(* Logix 5000 DataType export VMAC_DATA_INTERNAL; software revision 30.00 *)

TYPE Std_DiscreteAlarm :   // ALARM RESET
STRUCT
   AckC : BOOL;   // ALARM ACKNOWLEDGE
   LatchA : BOOL;   // ALARM LATCH
   DetectS : BOOL;   // ALARM DETECT
   BitS : BOOL;   // ALARM MISCOMPARE
   InhibitC : BOOL;   // ALARM INHIBIT
   Tmr : TIMER;   // ALARM Timer
END_STRUCT
END_TYPE

TYPE VMAC_DATA_INTERNAL :
STRUCT
   VMACOK : BOOL;
   CommsOK : BOOL;
   KeyOK : BOOL;
   KsInUse : BOOL;
   KsPrimeInUse : BOOL;
   EntryStatus : INT;
   NodeID : DINT;
   DestinationID : DINT;
   Counter : LINT;
   LastCounter : LINT;
   KeyID : LINT;
   VMAC_KEY : DINT[8];
   VMAC_CALC : DINT[8];
   VMAC_INPUT : DINT[8];
   DATA_INPUT : DINT[1600];
   DATA_VERIFIED : DINT[1600];
   VMAC_CTRL : VMAC;
   KeyAlarm : Std_DiscreteAlarm;
   ReplayAlarm : Std_DiscreteAlarm;
   InvalidAlarm : Std_DiscreteAlarm;
   NodeAlarm : Std_DiscreteAlarm;
   DestinationAlarm : Std_DiscreteAlarm;
   L_LES : L_LES;
   L_EQU : L_EQU;
   CommsTimer : TIMER;
END_STRUCT
END_TYPE

ADD_ON_INSTRUCTION D_SHR   (* revision 1.0 20170524, vendor Kenneth A. Fischer *)
// DINT bit shift right of the 32-bit argument Inp_A by Inp_B bits with paddding by zeros on the right
// Revision note:
// Rev1.0: 20170524 - Initial Release
VAR_IN_OUT
   Inp_A : DINT; {required}   // 64-bit Integer to be right circular rotated
END_VAR
VAR_INPUT
   Inp_B : INT; {required}   // Number of bits to shift
END_VAR
VAR_IN_OUT
   Out : DINT; {required}   // Result
END_VAR
VAR
   BSR_Cntrl : CONTROL := (LEN := 32);
   ONS : BOOL;
   Source_Bit : BOOL;
   Wrk_InpA : DINT[2];
END_VAR

ROUTINE Logic   (* ladder *)
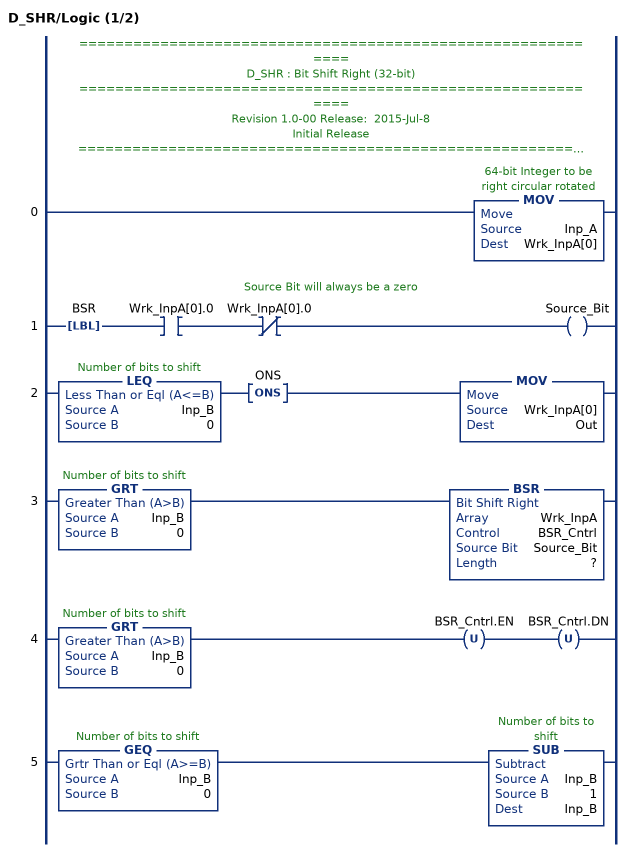
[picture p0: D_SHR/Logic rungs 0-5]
   // ============================================================
   // D_SHR : Bit Shift Right (32-bit)
   // ============================================================
   // Revision 1.0-00 Release:  2015-Jul-8
   // Initial Release
   // ============================================================
   // Performs a right bit shift of the 32-bit argument Inp_A by the
   // number of bits defined in the 16-bit argument Inp_B, with padding by zeros.
   0: MOV(Inp_A,Wrk_InpA[0]);
   // Source Bit will always be a zero
   1: LBL(BSR)XIC(Wrk_InpA[0].0)XIO(Wrk_InpA[0].0)OTE(Source_Bit);
   2: LEQ(Inp_B,0)ONS(ONS)MOV(Wrk_InpA[0],Out);
   3: GRT(Inp_B,0)BSR(Wrk_InpA,BSR_Cntrl,Source_Bit,?);
   4: GRT(Inp_B,0)OTU(BSR_Cntrl.EN)OTU(BSR_Cntrl.DN);
   5: GEQ(Inp_B,0)SUB(Inp_B,1,Inp_B);
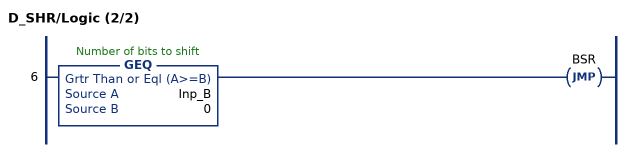
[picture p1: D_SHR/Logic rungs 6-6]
   6: GEQ(Inp_B,0)JMP(BSR);
END_ROUTINE
END_ADD_ON_INSTRUCTION

ADD_ON_INSTRUCTION D_ROTR   (* revision 1.0 20170524, vendor Kenneth A. Fischer *)
// DINT circular right shift (rotation) of the 32-bit argument Inp_A by Inp_B bits
// Revision note:
// Rev1.0: 20170524 - Initial Release
VAR_IN_OUT
   Inp_A : DINT; {required}   // 64-bit Integer to be right circular rotated
END_VAR
VAR_INPUT
   Inp_B : INT; {required}   // Number of Inp_A bit rotations
END_VAR
VAR_IN_OUT
   Out : DINT; {required}   // Result
END_VAR
VAR
   Wrk_InpA : DINT[2];
   BSR_Cntrl : CONTROL := (LEN := 32);
   Source_Bit : BOOL;
   ONS : BOOL;
END_VAR

ROUTINE Logic   (* ladder *)
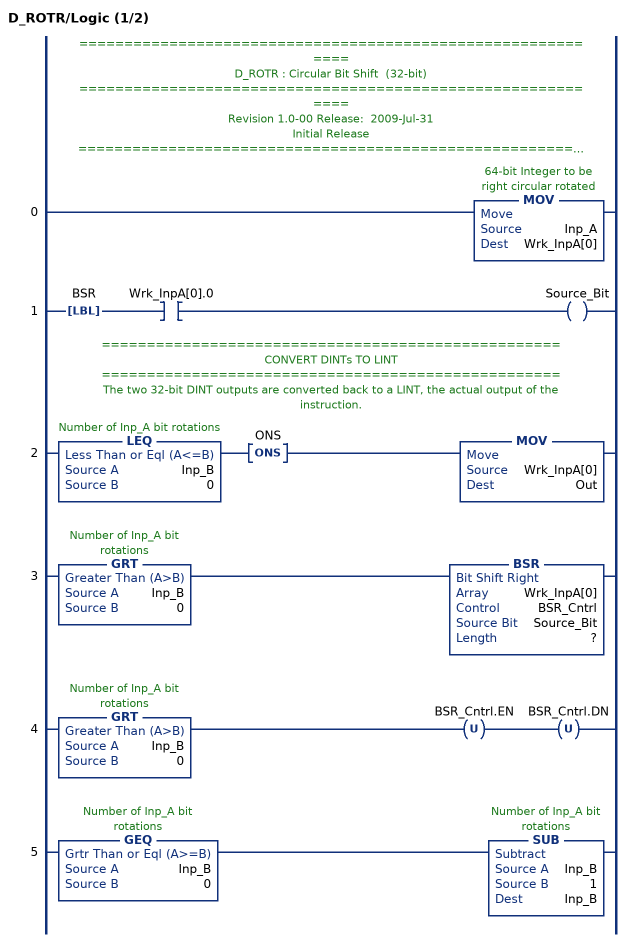
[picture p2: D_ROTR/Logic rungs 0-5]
   // ============================================================
   // D_ROTR : Circular Bit Shift  (32-bit)
   // ============================================================
   // Revision 1.0-00 Release:  2009-Jul-31
   // Initial Release
   // ============================================================
   // Performs a circular right shift rotation of the 32-bit argument Inp_A by the
   // number of bits defined in the 16-bit argument Inp_B.
   0: MOV(Inp_A,Wrk_InpA[0]);
   1: LBL(BSR)XIC(Wrk_InpA[0].0)OTE(Source_Bit);
   // ===================================================
   // CONVERT DINTs TO LINT
   // ===================================================
   // The two 32-bit DINT outputs are converted back to a LINT, the actual output of the instruction.
   2: LEQ(Inp_B,0)ONS(ONS)MOV(Wrk_InpA[0],Out);
   3: GRT(Inp_B,0)BSR(Wrk_InpA[0],BSR_Cntrl,Source_Bit,?);
   4: GRT(Inp_B,0)OTU(BSR_Cntrl.EN)OTU(BSR_Cntrl.DN);
   5: GEQ(Inp_B,0)SUB(Inp_B,1,Inp_B);
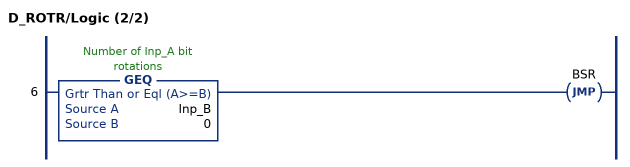
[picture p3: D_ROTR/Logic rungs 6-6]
   6: GEQ(Inp_B,0)JMP(BSR);
END_ROUTINE
END_ADD_ON_INSTRUCTION

ADD_ON_INSTRUCTION VMAC   (* revision 1.0 20170524, vendor Kenneth A. Fischer *)
// Variable Round MAC
// Revision note:
// Rev1.0: 20170524 - Initial Release
VAR_IN_OUT
   Inp_KEY : DINT[8]; {required}
   Inp_MSG : DINT[500]; {required}
END_VAR
VAR_INPUT
   Inp_LEN : DINT; {required}   // LENGTH INPUT OF MSG IN NUMBER OF DINTS
   Inp_ROUNDS : DINT; {required}
END_VAR
VAR_IN_OUT
   Out_VMAC : DINT[8]; {required}
        [0]   // HashBuffer_A
        [1]   // HashBuffer_B
        [2]   // HashBuffer_C
        [3]   // HashBuffer_D
        [4]   // HashBuffer_E
        [5]   // HashBuffer_F
        [6]   // HashBuffer_G
        [7]   // HashBuffer_H
END_VAR
VAR
   MajFunc : DINT;
   HashBuffer_H : DINT;
   HashBuffer_G : DINT;
   HashBuffer_F : DINT;
   HashBuffer_E : DINT;
   HashBuffer_D : DINT;
   HashBuffer_C : DINT;
   HashBuffer_B : DINT;
   HashBuffer_A : DINT;
   W : DINT[64];   // MESSAGE SCHEDULE
   tmp : DINT[20];
   T2 : DINT;
   T1 : DINT;
   t : INT;
   M : INT;   // MESSAGE INCREMENTS
   SigmaE : DINT;
   SigmaA : DINT;
   Sigma1 : DINT;
   Sigma0 : DINT;
   i : INT;
   x : INT;
   HashBufferInput_H : DINT;
   HashBufferInput_G : DINT;
   HashBufferInput_F : DINT;
   HashBufferInput_E : DINT;
   HashBufferInput_D : DINT;
   HashBufferInput_C : DINT;
   HashBufferInput_B : DINT;
   HashBufferInput_A : DINT;
   CondFunc : DINT;
   K : DINT[64];
   LENGTH_BITS : DINT;   // LENGTH OF MSG IN BITS
   LENGTH_MODULO : DINT;
   NUM_PADDING_BITS : DINT;   // NUMBER OF BITS NEEDED FOR PADDING
   NUM_PADDING_DINTS : DINT;   // NUMBER OF DINTS NEEDED FOR PADDING
   PADDING_COUNTER : DINT;
   TOTAL_MSG_LENGTH_MINUS_16 : DINT;
   D_ROTR : D_ROTR;
   D_SHR : D_SHR;
   ROUNDS : DINT;
   n : INT;
   KeyIndex : DINT;
   RotationIndex : DINT;
   IndexedKey : DINT;
END_VAR

ROUTINE Logic   (* ladder *)
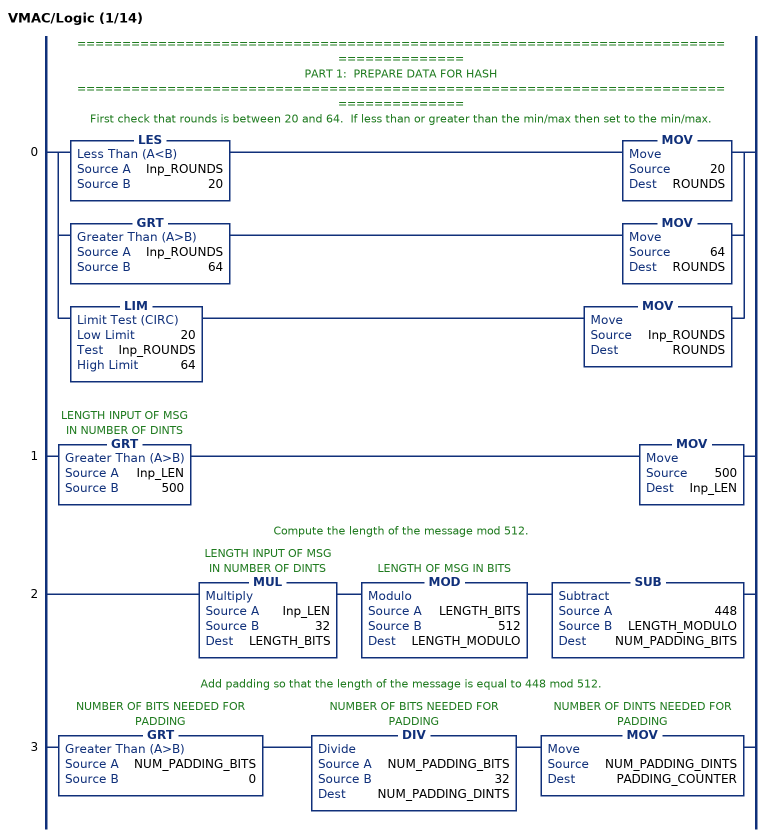
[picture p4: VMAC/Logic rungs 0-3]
   // ======================================================================================
   // PART 1:  PREPARE DATA FOR HASH
   // ======================================================================================
   // First check that rounds is between 20 and 64.  If less than or greater than the min/max then set to the min/max.
   0: [LES(Inp_ROUNDS,20) MOV(20,ROUNDS) ,GRT(Inp_ROUNDS,64) MOV(64,ROUNDS) ,LIM(20,Inp_ROUNDS,64) MOV(Inp_ROUNDS,ROUNDS) ];
   1: GRT(Inp_LEN,500)MOV(500,Inp_LEN);
   // Compute the length of the message mod 512.
   2: MUL(Inp_LEN,32,LENGTH_BITS)MOD(LENGTH_BITS,512,LENGTH_MODULO)SUB(448,LENGTH_MODULO,NUM_PADDING_BITS);
   // Add padding so that the length of the message is equal to 448 mod 512.
   3: GRT(NUM_PADDING_BITS,0)DIV(NUM_PADDING_BITS,32,NUM_PADDING_DINTS)MOV(NUM_PADDING_DINTS,PADDING_COUNTER);
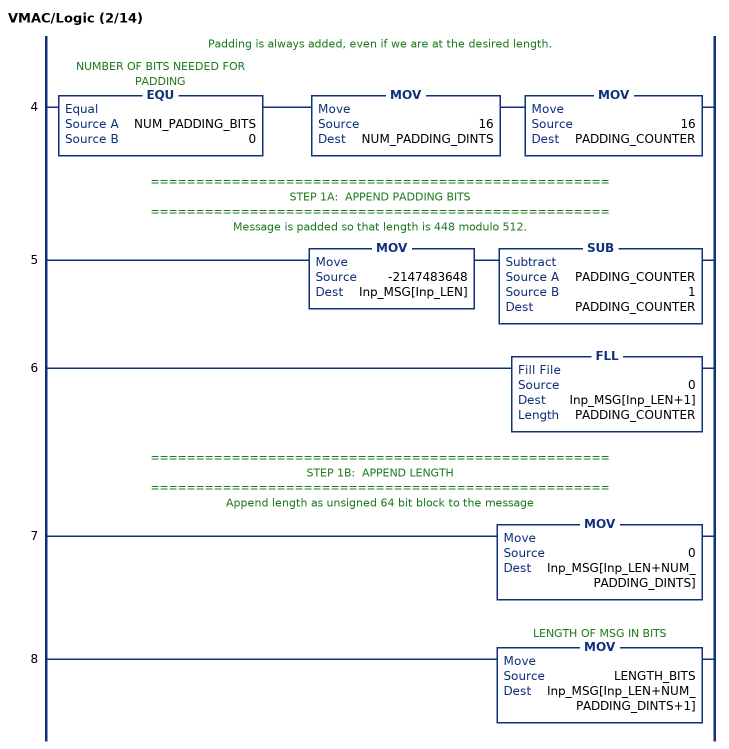
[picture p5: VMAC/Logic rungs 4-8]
   // Padding is always added, even if we are at the desired length.
   4: EQU(NUM_PADDING_BITS,0)MOV(16,NUM_PADDING_DINTS)MOV(16,PADDING_COUNTER);
   // ===================================================
   // STEP 1A:  APPEND PADDING BITS
   // ===================================================
   // Message is padded so that length is 448 modulo 512.
   5: MOV(-2147483648,Inp_MSG[Inp_LEN])SUB(PADDING_COUNTER,1,PADDING_COUNTER);
   6: FLL(0,Inp_MSG[Inp_LEN+1],PADDING_COUNTER);
   // ===================================================
   // STEP 1B:  APPEND LENGTH
   // ===================================================
   // Append length as unsigned 64 bit block to the message
   7: MOV(0,Inp_MSG[Inp_LEN+NUM_PADDING_DINTS]);
   8: MOV(LENGTH_BITS,Inp_MSG[Inp_LEN+NUM_PADDING_DINTS+1]);
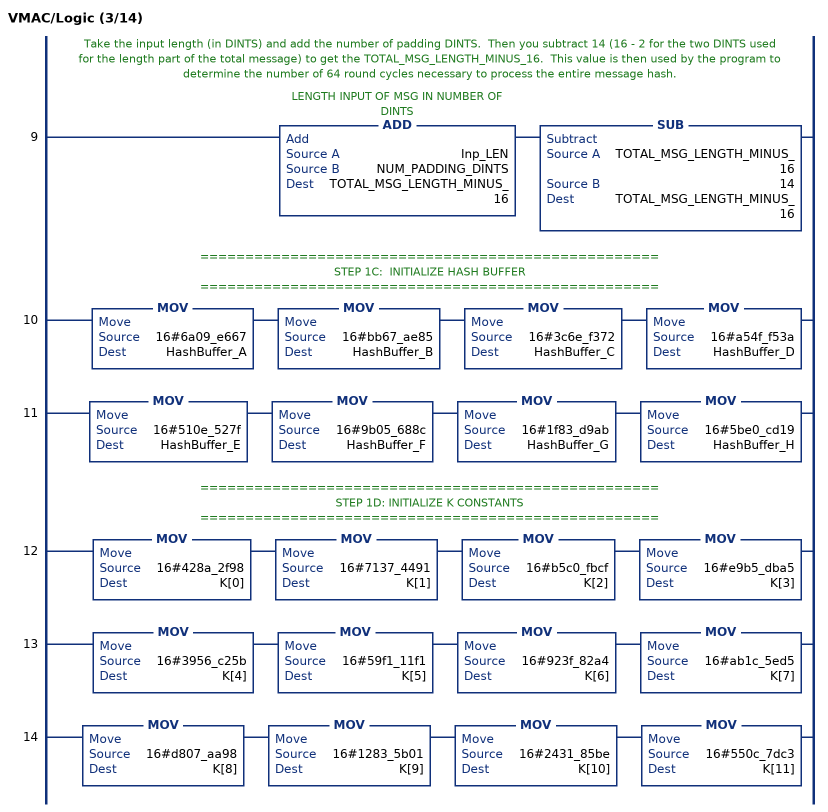
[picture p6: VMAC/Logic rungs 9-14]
   // Take the input length (in DINTS) and add the number of padding DINTS.  Then you subtract 14 (16 - 2 for the two DINTS used for the length part of the total message) to get the TOTAL_MSG_LENGTH_MINUS_16.  This value is then used by the program to determine the number of 64 round cycles necessary to process the entire message hash.
   9: ADD(Inp_LEN,NUM_PADDING_DINTS,TOTAL_MSG_LENGTH_MINUS_16)SUB(TOTAL_MSG_LENGTH_MINUS_16,14,TOTAL_MSG_LENGTH_MINUS_16);
   // ===================================================
   // STEP 1C:  INITIALIZE HASH BUFFER
   // ===================================================
   10: MOV(16#6a09_e667,HashBuffer_A)MOV(16#bb67_ae85,HashBuffer_B)MOV(16#3c6e_f372,HashBuffer_C)MOV(16#a54f_f53a,HashBuffer_D);
   11: MOV(16#510e_527f,HashBuffer_E)MOV(16#9b05_688c,HashBuffer_F)MOV(16#1f83_d9ab,HashBuffer_G)MOV(16#5be0_cd19,HashBuffer_H);
   // ===================================================
   // STEP 1D: INITIALIZE K CONSTANTS
   // ===================================================
   12: MOV(16#428a_2f98,K[0])MOV(16#7137_4491,K[1])MOV(16#b5c0_fbcf,K[2])MOV(16#e9b5_dba5,K[3]);
   13: MOV(16#3956_c25b,K[4])MOV(16#59f1_11f1,K[5])MOV(16#923f_82a4,K[6])MOV(16#ab1c_5ed5,K[7]);
   14: MOV(16#d807_aa98,K[8])MOV(16#1283_5b01,K[9])MOV(16#2431_85be,K[10])MOV(16#550c_7dc3,K[11]);
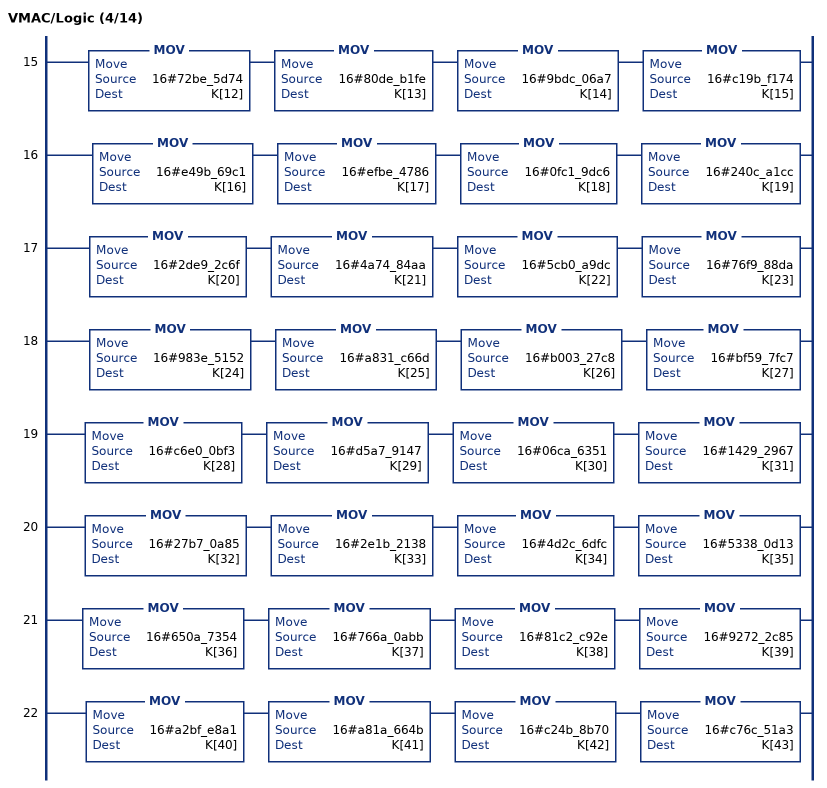
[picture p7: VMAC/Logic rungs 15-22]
   15: MOV(16#72be_5d74,K[12])MOV(16#80de_b1fe,K[13])MOV(16#9bdc_06a7,K[14])MOV(16#c19b_f174,K[15]);
   16: MOV(16#e49b_69c1,K[16])MOV(16#efbe_4786,K[17])MOV(16#0fc1_9dc6,K[18])MOV(16#240c_a1cc,K[19]);
   17: MOV(16#2de9_2c6f,K[20])MOV(16#4a74_84aa,K[21])MOV(16#5cb0_a9dc,K[22])MOV(16#76f9_88da,K[23]);
   18: MOV(16#983e_5152,K[24])MOV(16#a831_c66d,K[25])MOV(16#b003_27c8,K[26])MOV(16#bf59_7fc7,K[27]);
   19: MOV(16#c6e0_0bf3,K[28])MOV(16#d5a7_9147,K[29])MOV(16#06ca_6351,K[30])MOV(16#1429_2967,K[31]);
   20: MOV(16#27b7_0a85,K[32])MOV(16#2e1b_2138,K[33])MOV(16#4d2c_6dfc,K[34])MOV(16#5338_0d13,K[35]);
   21: MOV(16#650a_7354,K[36])MOV(16#766a_0abb,K[37])MOV(16#81c2_c92e,K[38])MOV(16#9272_2c85,K[39]);
   22: MOV(16#a2bf_e8a1,K[40])MOV(16#a81a_664b,K[41])MOV(16#c24b_8b70,K[42])MOV(16#c76c_51a3,K[43]);
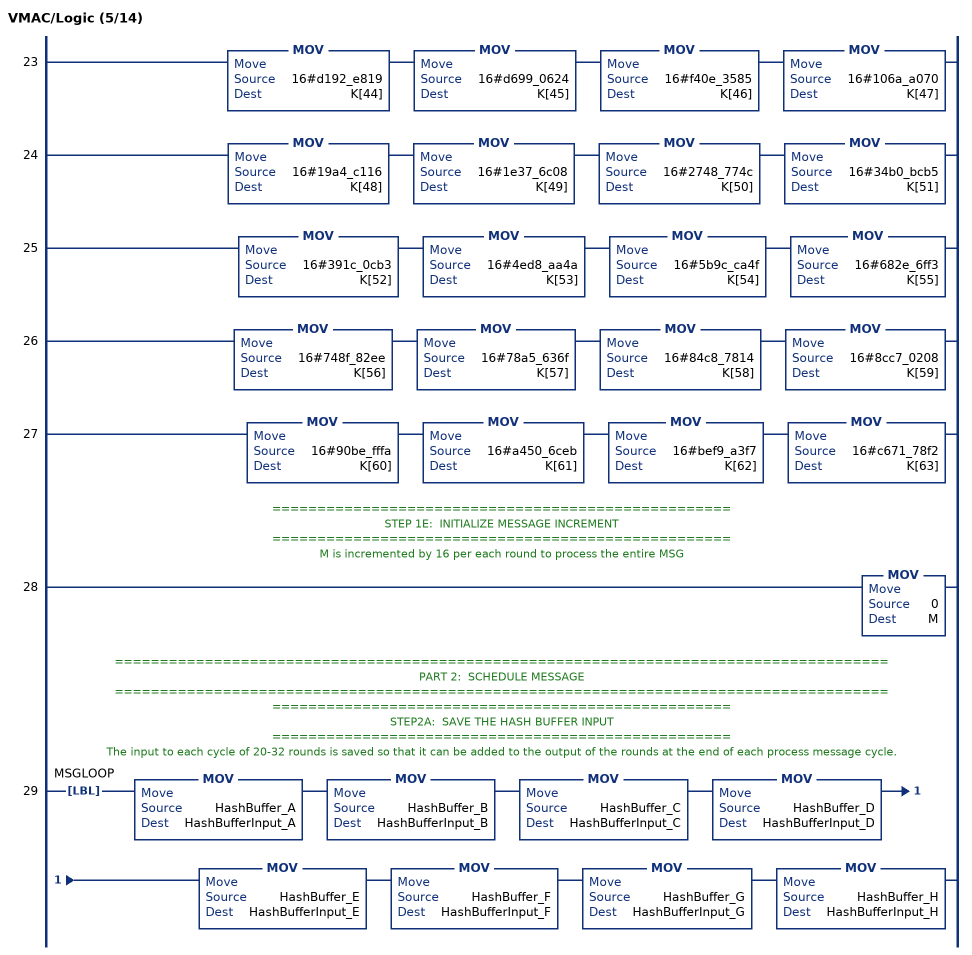
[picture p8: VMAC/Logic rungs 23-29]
   23: MOV(16#d192_e819,K[44])MOV(16#d699_0624,K[45])MOV(16#f40e_3585,K[46])MOV(16#106a_a070,K[47]);
   24: MOV(16#19a4_c116,K[48])MOV(16#1e37_6c08,K[49])MOV(16#2748_774c,K[50])MOV(16#34b0_bcb5,K[51]);
   25: MOV(16#391c_0cb3,K[52])MOV(16#4ed8_aa4a,K[53])MOV(16#5b9c_ca4f,K[54])MOV(16#682e_6ff3,K[55]);
   26: MOV(16#748f_82ee,K[56])MOV(16#78a5_636f,K[57])MOV(16#84c8_7814,K[58])MOV(16#8cc7_0208,K[59]);
   27: MOV(16#90be_fffa,K[60])MOV(16#a450_6ceb,K[61])MOV(16#bef9_a3f7,K[62])MOV(16#c671_78f2,K[63]);
   // ===================================================
   // STEP 1E:  INITIALIZE MESSAGE INCREMENT
   // ===================================================
   // M is incremented by 16 per each round to process the entire MSG
   28: MOV(0,M);
   // ======================================================================================
   // PART 2:  SCHEDULE MESSAGE
   // ======================================================================================
   // ===================================================
   // STEP2A:  SAVE THE HASH BUFFER INPUT
   // ===================================================
   // The input to each cycle of 20-32 rounds is saved so that it can be added to the output of the rounds at the end of each process message cycle.
   29: LBL(MSGLOOP)MOV(HashBuffer_A,HashBufferInput_A)MOV(HashBuffer_B,HashBufferInput_B)MOV(HashBuffer_C,HashBufferInput_C)MOV(HashBuffer_D,HashBufferInput_D)MOV(HashBuffer_E,HashBufferInput_E)MOV(HashBuffer_F,HashBufferInput_F)MOV(HashBuffer_G,HashBufferInput_G)MOV(HashBuffer_H,HashBufferInput_H);
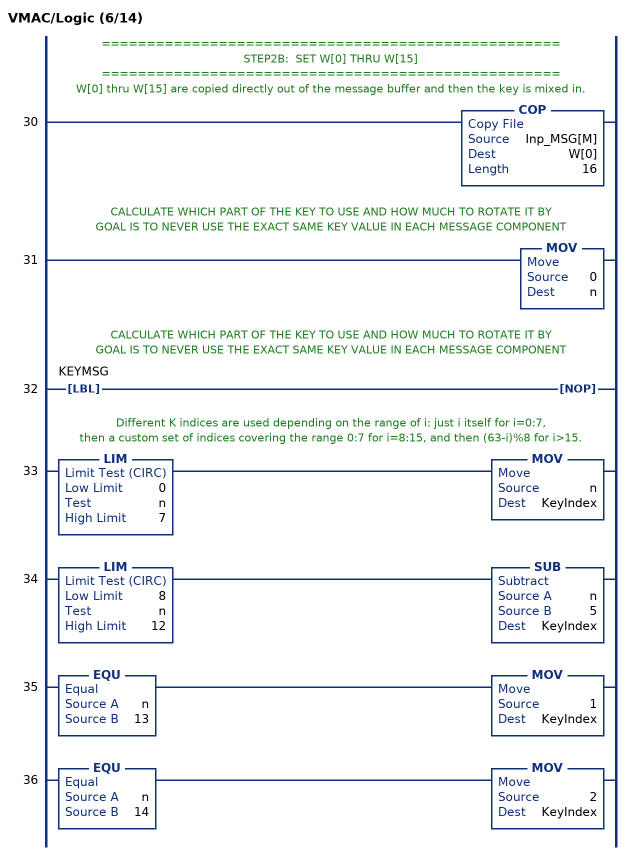
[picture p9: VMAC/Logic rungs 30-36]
   // ===================================================
   // STEP2B:  SET W[0] THRU W[15]
   // ===================================================
   // W[0] thru W[15] are copied directly out of the message buffer and then the key is mixed in.
   30: COP(Inp_MSG[M],W[0],16);
   // CALCULATE WHICH PART OF THE KEY TO USE AND HOW MUCH TO ROTATE IT BY
   // GOAL IS TO NEVER USE THE EXACT SAME KEY VALUE IN EACH MESSAGE COMPONENT
   31: MOV(0,n);
   // CALCULATE WHICH PART OF THE KEY TO USE AND HOW MUCH TO ROTATE IT BY
   // GOAL IS TO NEVER USE THE EXACT SAME KEY VALUE IN EACH MESSAGE COMPONENT
   32: LBL(KEYMSG)NOP();
   // Different K indices are used depending on the range of i: just i itself for i=0:7,
   // then a custom set of indices covering the range 0:7 for i=8:15, and then (63-i)%8 for i>15.
   33: LIM(0,n,7)MOV(n,KeyIndex);
   34: LIM(8,n,12)SUB(n,5,KeyIndex);
   35: EQU(n,13)MOV(1,KeyIndex);
   36: EQU(n,14)MOV(2,KeyIndex);
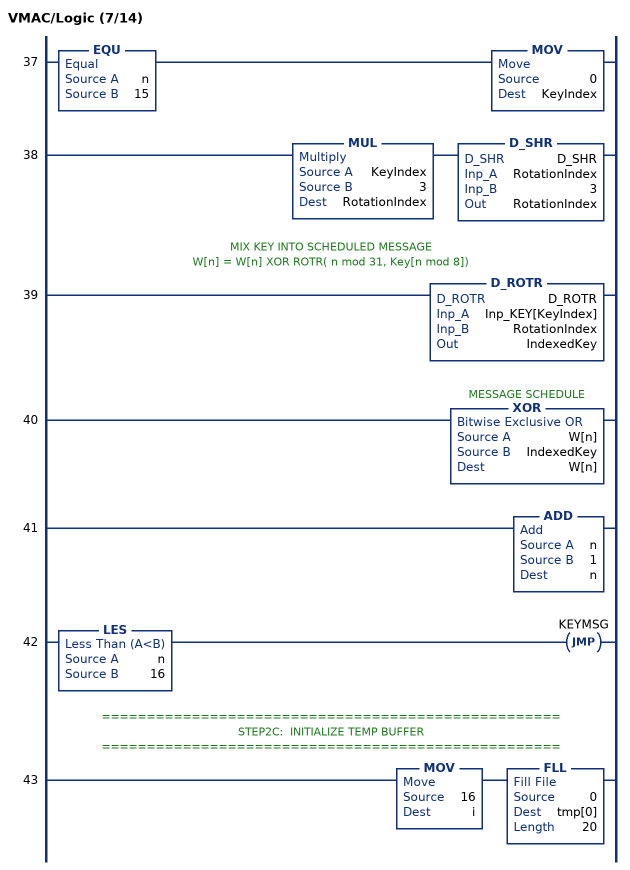
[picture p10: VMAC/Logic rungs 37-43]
   37: EQU(n,15)MOV(0,KeyIndex);
   38: MUL(KeyIndex,3,RotationIndex)D_SHR(D_SHR,RotationIndex,3,RotationIndex);
   // MIX KEY INTO SCHEDULED MESSAGE
   // W[n] = W[n] XOR ROTR( n mod 31, Key[n mod 8])
   39: D_ROTR(D_ROTR,Inp_KEY[KeyIndex],RotationIndex,IndexedKey);
   40: XOR(W[n],IndexedKey,W[n]);
   41: ADD(n,1,n);
   42: LES(n,16)JMP(KEYMSG);
   // ===================================================
   // STEP2C:  INITIALIZE TEMP BUFFER
   // ===================================================
   43: MOV(16,i)FLL(0,tmp[0],20);
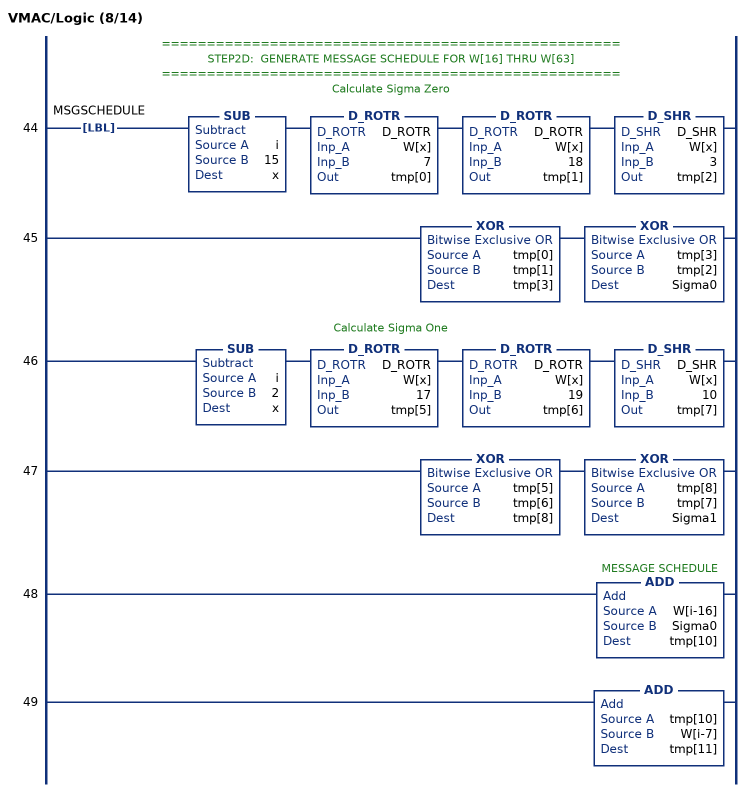
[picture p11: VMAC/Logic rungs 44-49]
   // ===================================================
   // STEP2D:  GENERATE MESSAGE SCHEDULE FOR W[16] THRU W[63]
   // ===================================================
   // Calculate Sigma Zero
   44: LBL(MSGSCHEDULE)SUB(i,15,x)D_ROTR(D_ROTR,W[x],7,tmp[0])D_ROTR(D_ROTR,W[x],18,tmp[1])D_SHR(D_SHR,W[x],3,tmp[2]);
   45: XOR(tmp[0],tmp[1],tmp[3])XOR(tmp[3],tmp[2],Sigma0);
   // Calculate Sigma One
   46: SUB(i,2,x)D_ROTR(D_ROTR,W[x],17,tmp[5])D_ROTR(D_ROTR,W[x],19,tmp[6])D_SHR(D_SHR,W[x],10,tmp[7]);
   47: XOR(tmp[5],tmp[6],tmp[8])XOR(tmp[8],tmp[7],Sigma1);
   48: ADD(W[i-16],Sigma0,tmp[10]);
   49: ADD(tmp[10],W[i-7],tmp[11]);
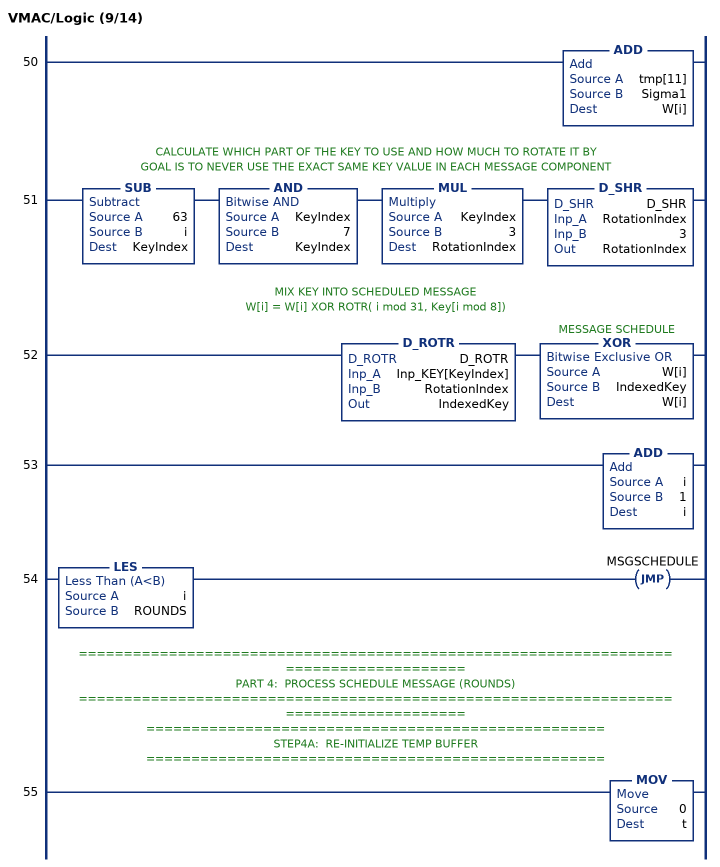
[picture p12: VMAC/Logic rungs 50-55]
   50: ADD(tmp[11],Sigma1,W[i]);
   // CALCULATE WHICH PART OF THE KEY TO USE AND HOW MUCH TO ROTATE IT BY
   // GOAL IS TO NEVER USE THE EXACT SAME KEY VALUE IN EACH MESSAGE COMPONENT
   51: SUB(63,i,KeyIndex)AND(KeyIndex,7,KeyIndex)MUL(KeyIndex,3,RotationIndex)D_SHR(D_SHR,RotationIndex,3,RotationIndex);
   // MIX KEY INTO SCHEDULED MESSAGE
   // W[i] = W[i] XOR ROTR( i mod 31, Key[i mod 8])
   52: D_ROTR(D_ROTR,Inp_KEY[KeyIndex],RotationIndex,IndexedKey)XOR(W[i],IndexedKey,W[i]);
   53: ADD(i,1,i);
   54: LES(i,ROUNDS)JMP(MSGSCHEDULE);
   // ======================================================================================
   // PART 4:  PROCESS SCHEDULE MESSAGE (ROUNDS)
   // ======================================================================================
   // ===================================================
   // STEP4A:  RE-INITIALIZE TEMP BUFFER
   // ===================================================
   55: MOV(0,t);
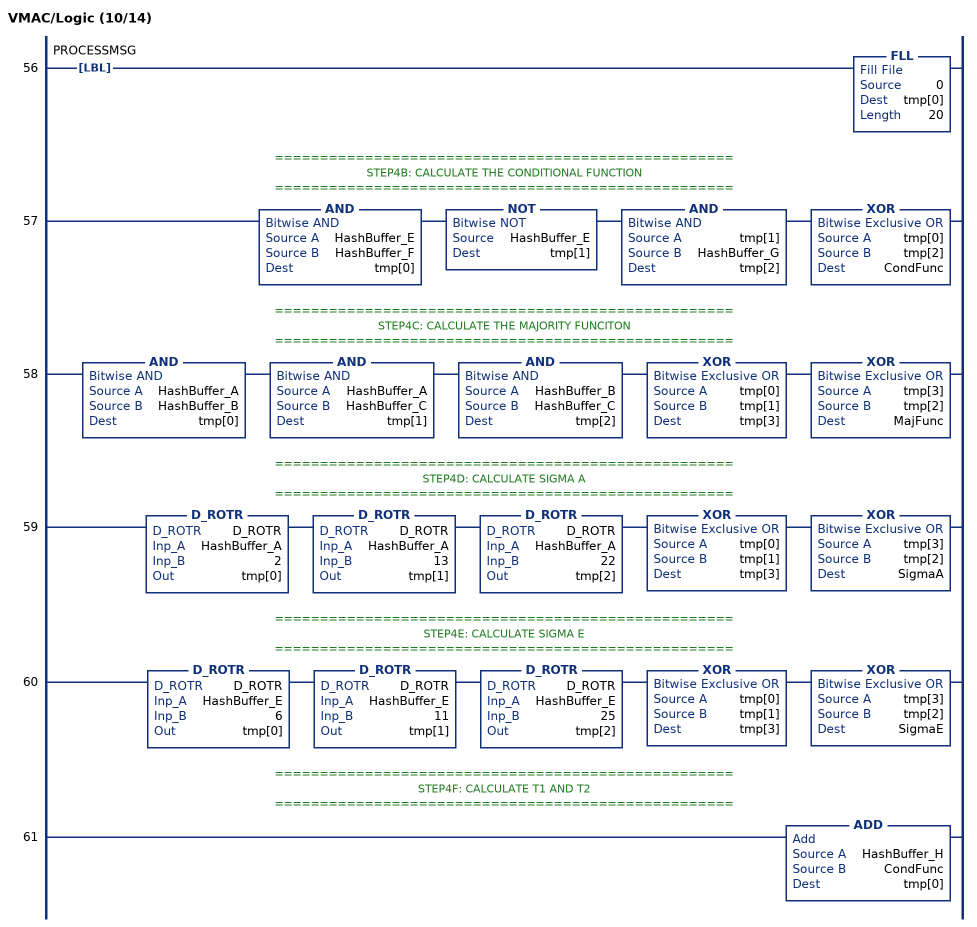
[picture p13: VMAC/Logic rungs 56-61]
   56: LBL(PROCESSMSG)FLL(0,tmp[0],20);
   // ===================================================
   // STEP4B: CALCULATE THE CONDITIONAL FUNCTION
   // ===================================================
   57: AND(HashBuffer_E,HashBuffer_F,tmp[0])NOT(HashBuffer_E,tmp[1])AND(tmp[1],HashBuffer_G,tmp[2])XOR(tmp[0],tmp[2],CondFunc);
   // ===================================================
   // STEP4C: CALCULATE THE MAJORITY FUNCITON
   // ===================================================
   58: AND(HashBuffer_A,HashBuffer_B,tmp[0])AND(HashBuffer_A,HashBuffer_C,tmp[1])AND(HashBuffer_B,HashBuffer_C,tmp[2])XOR(tmp[0],tmp[1],tmp[3])XOR(tmp[3],tmp[2],MajFunc);
   // ===================================================
   // STEP4D: CALCULATE SIGMA A
   // ===================================================
   59: D_ROTR(D_ROTR,HashBuffer_A,2,tmp[0])D_ROTR(D_ROTR,HashBuffer_A,13,tmp[1])D_ROTR(D_ROTR,HashBuffer_A,22,tmp[2])XOR(tmp[0],tmp[1],tmp[3])XOR(tmp[3],tmp[2],SigmaA);
   // ===================================================
   // STEP4E: CALCULATE SIGMA E
   // ===================================================
   60: D_ROTR(D_ROTR,HashBuffer_E,6,tmp[0])D_ROTR(D_ROTR,HashBuffer_E,11,tmp[1])D_ROTR(D_ROTR,HashBuffer_E,25,tmp[2])XOR(tmp[0],tmp[1],tmp[3])XOR(tmp[3],tmp[2],SigmaE);
   // ===================================================
   // STEP4F: CALCULATE T1 AND T2
   // ===================================================
   61: ADD(HashBuffer_H,CondFunc,tmp[0]);
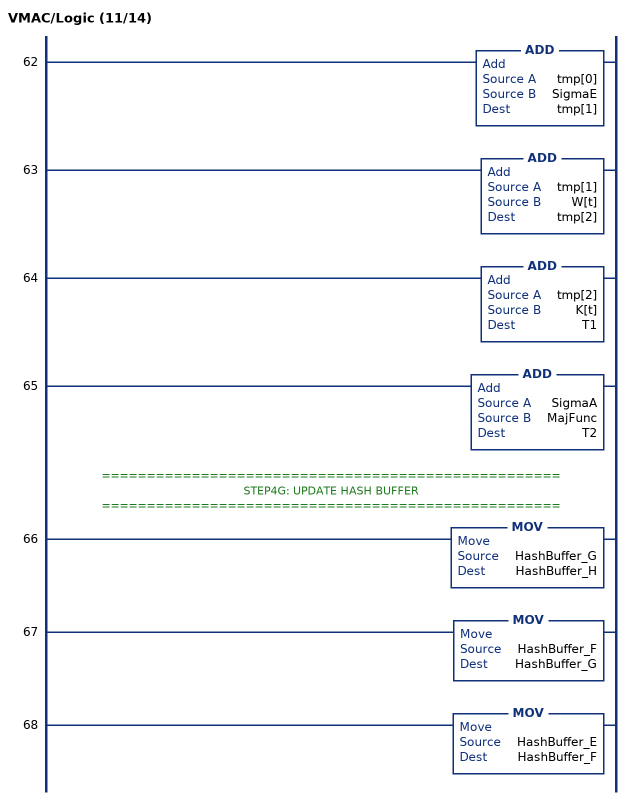
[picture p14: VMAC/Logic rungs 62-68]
   62: ADD(tmp[0],SigmaE,tmp[1]);
   63: ADD(tmp[1],W[t],tmp[2]);
   64: ADD(tmp[2],K[t],T1);
   65: ADD(SigmaA,MajFunc,T2);
   // ===================================================
   // STEP4G: UPDATE HASH BUFFER
   // ===================================================
   66: MOV(HashBuffer_G,HashBuffer_H);
   67: MOV(HashBuffer_F,HashBuffer_G);
   68: MOV(HashBuffer_E,HashBuffer_F);
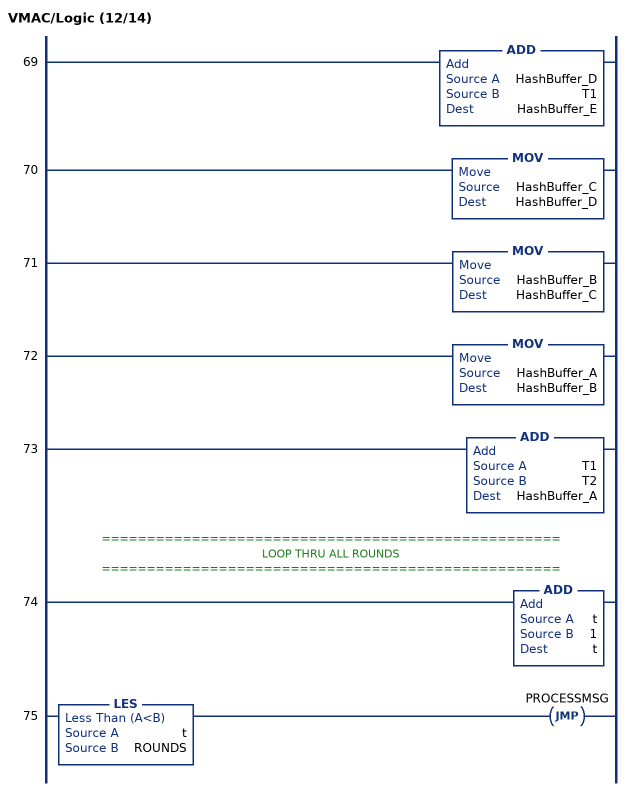
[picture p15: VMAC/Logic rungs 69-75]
   69: ADD(HashBuffer_D,T1,HashBuffer_E);
   70: MOV(HashBuffer_C,HashBuffer_D);
   71: MOV(HashBuffer_B,HashBuffer_C);
   72: MOV(HashBuffer_A,HashBuffer_B);
   73: ADD(T1,T2,HashBuffer_A);
   // ===================================================
   // LOOP THRU ALL ROUNDS
   // ===================================================
   74: ADD(t,1,t);
   75: LES(t,ROUNDS)JMP(PROCESSMSG);
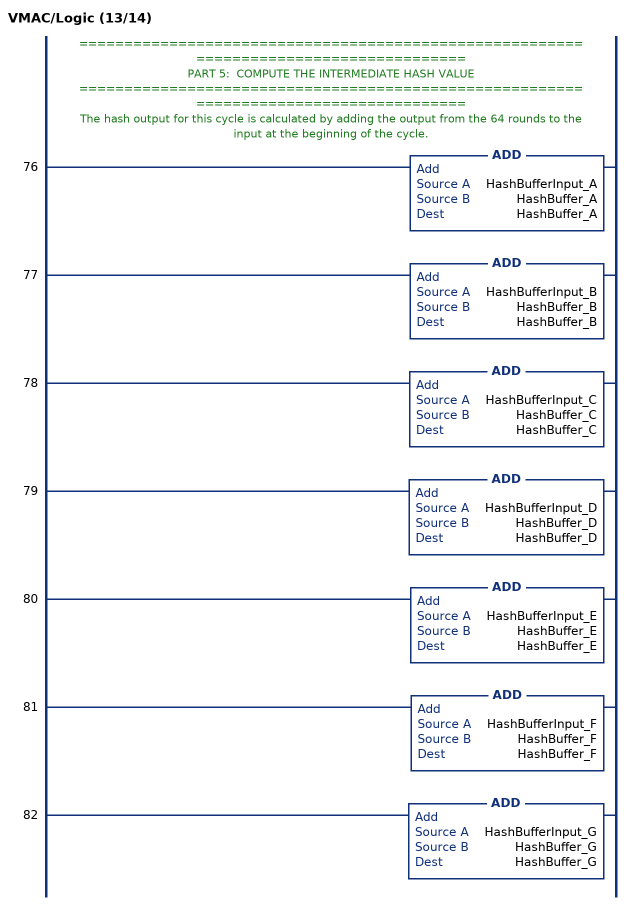
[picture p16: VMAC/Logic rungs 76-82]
   // ======================================================================================
   // PART 5:  COMPUTE THE INTERMEDIATE HASH VALUE
   // ======================================================================================
   // The hash output for this cycle is calculated by adding the output from the 64 rounds to the input at the beginning of the cycle.
   76: ADD(HashBufferInput_A,HashBuffer_A,HashBuffer_A);
   77: ADD(HashBufferInput_B,HashBuffer_B,HashBuffer_B);
   78: ADD(HashBufferInput_C,HashBuffer_C,HashBuffer_C);
   79: ADD(HashBufferInput_D,HashBuffer_D,HashBuffer_D);
   80: ADD(HashBufferInput_E,HashBuffer_E,HashBuffer_E);
   81: ADD(HashBufferInput_F,HashBuffer_F,HashBuffer_F);
   82: ADD(HashBufferInput_G,HashBuffer_G,HashBuffer_G);
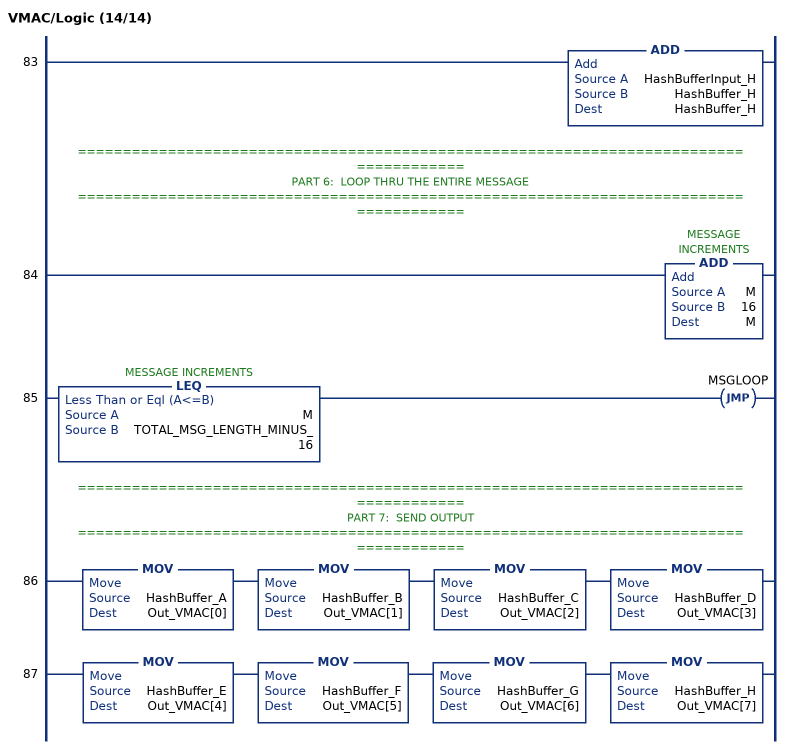
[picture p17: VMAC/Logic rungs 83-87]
   83: ADD(HashBufferInput_H,HashBuffer_H,HashBuffer_H);
   // ======================================================================================
   // PART 6:  LOOP THRU THE ENTIRE MESSAGE
   // ======================================================================================
   84: ADD(M,16,M);
   85: LEQ(M,TOTAL_MSG_LENGTH_MINUS_16)JMP(MSGLOOP);
   // ======================================================================================
   // PART 7:  SEND OUTPUT
   // ======================================================================================
   86: MOV(HashBuffer_A,Out_VMAC[0])MOV(HashBuffer_B,Out_VMAC[1])MOV(HashBuffer_C,Out_VMAC[2])MOV(HashBuffer_D,Out_VMAC[3]);
   87: MOV(HashBuffer_E,Out_VMAC[4])MOV(HashBuffer_F,Out_VMAC[5])MOV(HashBuffer_G,Out_VMAC[6])MOV(HashBuffer_H,Out_VMAC[7]);
END_ROUTINE
END_ADD_ON_INSTRUCTION

ADD_ON_INSTRUCTION L_EQU   (* revision 1.0 01 Release, vendor Rockwell Automation, ExecuteEnableInFalse *)
// Equal (64-bit)
// Revision note:
// Deleted unused Local Tag
// Help:
// This instruction compares two LINT (64-bit signed integer) variables.
// If Inp_A is equal to Inp_B, EnableOut and Out are set to true (1).
// Otherwise EnableOut and Out are cleared to false (0).
VAR_IN_OUT
   Inp_A : LINT; {required}   // Input A
   Inp_B : LINT; {required}   // Input B
END_VAR
VAR_OUTPUT
   Out : BOOL; {access Read Only, visible}   // TRUE if Inp_A is greater than or equal to Inp_B
END_VAR
VAR
   Wrk_Inp_B : DINT[2];   // 32-bit portions of Input B
   Wrk_Inp_A : DINT[2];   // 32-bit portions of Input A
END_VAR

ROUTINE EnableInFalse   (* ladder *)
// If rung is false, clear output "Out"
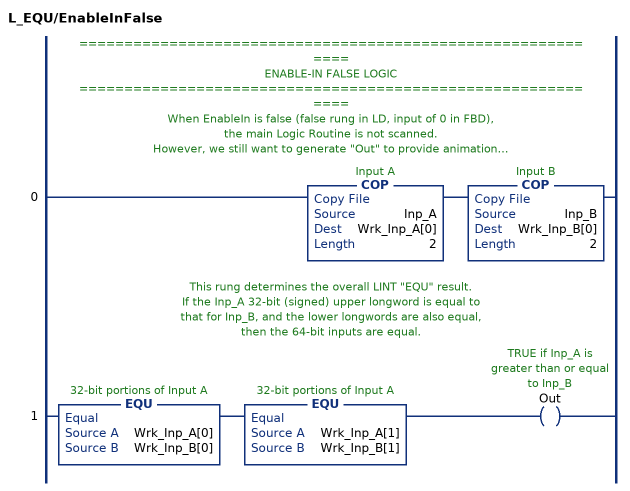
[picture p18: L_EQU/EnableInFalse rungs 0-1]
   // ============================================================
   // ENABLE-IN FALSE LOGIC
   // ============================================================
   // When EnableIn is false (false rung in LD, input of 0 in FBD),
   // the main Logic Routine is not scanned.
   // However, we still want to generate "Out" to provide animation!
   // ===================================================
   // CONVERT LINTs TO DINTs
   // ===================================================
   // These COPies take the input LINTs and break them into a
   // pair of DINTs each.  If the corresponding DINTs (high-order and high-order,
   // and low-order and low-order) are equal, then the input LINTs are equal.
   0: COP(Inp_A,Wrk_Inp_A[0],2)COP(Inp_B,Wrk_Inp_B[0],2);
   // This rung determines the overall LINT "EQU" result.
   // If the Inp_A 32-bit (signed) upper longword is equal to
   // that for Inp_B, and the lower longwords are also equal,
   // then the 64-bit inputs are equal.
   1: EQU(Wrk_Inp_A[0],Wrk_Inp_B[0])EQU(Wrk_Inp_A[1],Wrk_Inp_B[1])OTE(Out);
END_ROUTINE

ROUTINE Logic   (* ladder *)
// Compare inputs and output TRUE if they are equal
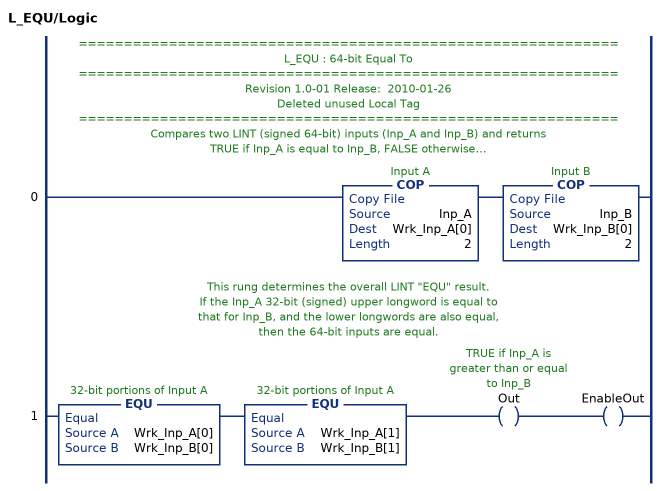
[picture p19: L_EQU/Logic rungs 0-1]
   // ============================================================
   // L_EQU : 64-bit Equal To
   // ============================================================
   // Revision 1.0-01 Release:  2010-01-26
   // Deleted unused Local Tag
   // ============================================================
   // Compares two LINT (signed 64-bit) inputs (Inp_A and Inp_B) and returns
   // TRUE if Inp_A is equal to Inp_B, FALSE otherwise.
   // This instruction breaks each LINT inputs into two DINTs
   // (32 bit signed each) to do the comparison.
   // ===================================================
   // CONVERT LINTs TO DINTs
   // ===================================================
   // These COPies take the input LINTs and break them into a
   // pair of DINTs each.  If the corresponding DINTs (high-order and high-order,
   // and low-order and low-order) are equal, then the input LINTs are equal.
   0: COP(Inp_A,Wrk_Inp_A[0],2)COP(Inp_B,Wrk_Inp_B[0],2);
   // This rung determines the overall LINT "EQU" result.
   // If the Inp_A 32-bit (signed) upper longword is equal to
   // that for Inp_B, and the lower longwords are also equal,
   // then the 64-bit inputs are equal.
   1: EQU(Wrk_Inp_A[0],Wrk_Inp_B[0])EQU(Wrk_Inp_A[1],Wrk_Inp_B[1])OTE(Out)OTE(EnableOut);
END_ROUTINE
END_ADD_ON_INSTRUCTION

ADD_ON_INSTRUCTION L_LES   (* revision 1.1 20170624, vendor Ken Fischer, NSWCPD, C516, ExecuteEnableInFalse *)
// Less Than (64-bit)
// Revision note:
// Rev1.1:  20170624 - Corrected comment on the Out bit
// Help:
// This instruction compares two LINT (64-bit signed integer) variables.
// If Inp_A is less than Inp_B, EnableOut and Out are set to true (1).
// Otherwise EnableOut and Out are cleared to false (0).
VAR_IN_OUT
   Inp_A : LINT; {required}   // Input A
   Inp_B : LINT; {required}   // Input B
END_VAR
VAR_OUTPUT
   Out : BOOL; {access Read Only, visible}   // TRUE if Inp_A is less than Inp_B
END_VAR
VAR
   Wrk_Inp_B : DINT[4];   // 32-bit portions of Input B
   Wrk_Inp_A : DINT[4];   // 32-bit portions of Input A
END_VAR

ROUTINE EnableInFalse   (* ladder *)
// If rung is false, clear output "Out"
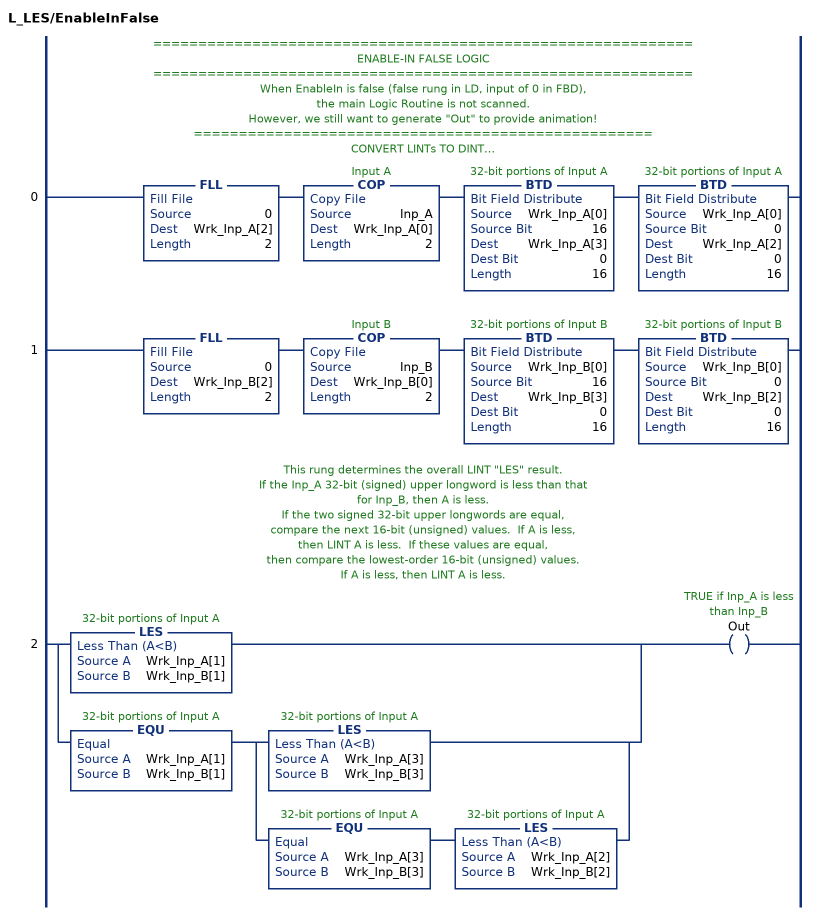
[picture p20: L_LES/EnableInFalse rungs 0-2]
   // ============================================================
   // ENABLE-IN FALSE LOGIC
   // ============================================================
   // When EnableIn is false (false rung in LD, input of 0 in FBD),
   // the main Logic Routine is not scanned.
   // However, we still want to generate "Out" to provide animation!
   // ===================================================
   // CONVERT LINTs TO DINTs
   // ===================================================
   // These COPies and BTDs take the input LINTs and break them into a
   // pair of DINTs each, then take the low-order signed DINT and breaks it
   // further into two 16-bit values so we can do unsigned compares on them.
   // Logix V17 has a LINT data type, but math instructions
   // (and AOI Input and Output Parameters) don't support LINT.
   0: FLL(0,Wrk_Inp_A[2],2)COP(Inp_A,Wrk_Inp_A[0],2)BTD(Wrk_Inp_A[0],16,Wrk_Inp_A[3],0,16)BTD(Wrk_Inp_A[0],0,Wrk_Inp_A[2],0,16);
   1: FLL(0,Wrk_Inp_B[2],2)COP(Inp_B,Wrk_Inp_B[0],2)BTD(Wrk_Inp_B[0],16,Wrk_Inp_B[3],0,16)BTD(Wrk_Inp_B[0],0,Wrk_Inp_B[2],0,16);
   // This rung determines the overall LINT "LES" result.
   // If the Inp_A 32-bit (signed) upper longword is less than that
   // for Inp_B, then A is less.
   // If the two signed 32-bit upper longwords are equal,
   // compare the next 16-bit (unsigned) values.  If A is less,
   // then LINT A is less.  If these values are equal,
   // then compare the lowest-order 16-bit (unsigned) values.
   // If A is less, then LINT A is less.
   2: [LES(Wrk_Inp_A[1],Wrk_Inp_B[1]) ,EQU(Wrk_Inp_A[1],Wrk_Inp_B[1]) [LES(Wrk_Inp_A[3],Wrk_Inp_B[3]) ,EQU(Wrk_Inp_A[3],Wrk_Inp_B[3]) LES(Wrk_Inp_A[2],Wrk_Inp_B[2]) ] ]OTE(Out);
END_ROUTINE

ROUTINE Logic   (* ladder *)
// Compare inputs and output TRUE if Inp_A < Inp_B
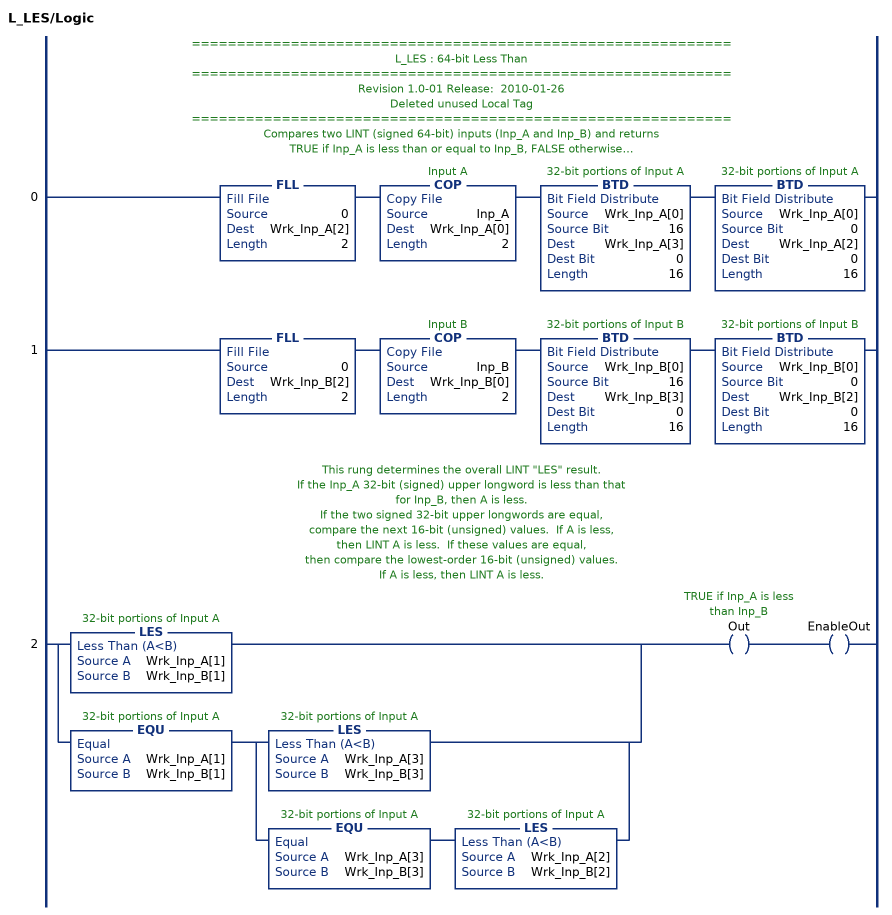
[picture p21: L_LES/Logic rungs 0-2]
   // ============================================================
   // L_LES : 64-bit Less Than
   // ============================================================
   // Revision 1.0-01 Release:  2010-01-26
   // Deleted unused Local Tag
   // ============================================================
   // Compares two LINT (signed 64-bit) inputs (Inp_A and Inp_B) and returns
   // TRUE if Inp_A is less than or equal to Inp_B, FALSE otherwise.
   // This instruction breaks the LINT inputs into three DINTs
   // (32 bit signed, 16 bit unsigned and 16 bit unsigned) to do the comparison.
   // ===================================================
   // CONVERT LINTs TO DINTs
   // ===================================================
   // These COPies and BTDs take the input LINTs and break them into a
   // pair of DINTs each, then take the low-order signed DINT and breaks it
   // further into two 16-bit values so we can do unsigned compares on them.
   // Logix V17 has a LINT data type, but math instructions
   // (and AOI Input and Output Parameters) don't support LINT.
   0: FLL(0,Wrk_Inp_A[2],2)COP(Inp_A,Wrk_Inp_A[0],2)BTD(Wrk_Inp_A[0],16,Wrk_Inp_A[3],0,16)BTD(Wrk_Inp_A[0],0,Wrk_Inp_A[2],0,16);
   1: FLL(0,Wrk_Inp_B[2],2)COP(Inp_B,Wrk_Inp_B[0],2)BTD(Wrk_Inp_B[0],16,Wrk_Inp_B[3],0,16)BTD(Wrk_Inp_B[0],0,Wrk_Inp_B[2],0,16);
   // This rung determines the overall LINT "LES" result.
   // If the Inp_A 32-bit (signed) upper longword is less than that
   // for Inp_B, then A is less.
   // If the two signed 32-bit upper longwords are equal,
   // compare the next 16-bit (unsigned) values.  If A is less,
   // then LINT A is less.  If these values are equal,
   // then compare the lowest-order 16-bit (unsigned) values.
   // If A is less, then LINT A is less.
   2: [LES(Wrk_Inp_A[1],Wrk_Inp_B[1]) ,EQU(Wrk_Inp_A[1],Wrk_Inp_B[1]) [LES(Wrk_Inp_A[3],Wrk_Inp_B[3]) ,EQU(Wrk_Inp_A[3],Wrk_Inp_B[3]) LES(Wrk_Inp_A[2],Wrk_Inp_B[2]) ] ]OTE(Out)OTE(EnableOut);
END_ROUTINE
END_ADD_ON_INSTRUCTION
